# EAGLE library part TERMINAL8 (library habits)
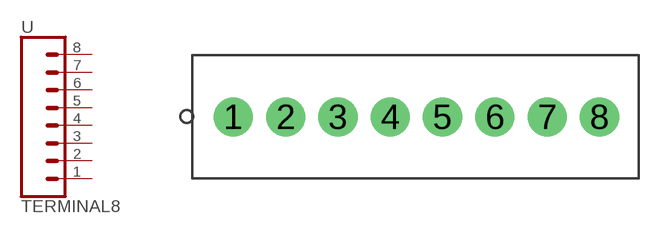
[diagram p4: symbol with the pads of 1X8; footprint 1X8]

Designator prefix -

## TERMINAL8  [1X8]
1  1  pas
2  2  pas
3  3  pas
4  4  pas
5  5  pas
6  6  pas
7  7  pas
8  8  pas

## Footprint 1X8 (pad centres in mm)
Plated Through Hole -16 Pin Specifications: Pin count:16 Pin pitch:0.1" Example device(s): CONN_16
drill 1 pad 1.9: 1 0,0; 2 2.54,0; 3 5.08,0; 4 7.62,0; 5 10.16,0; 6 12.7,0; 7 15.24,0; 8 17.78,0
